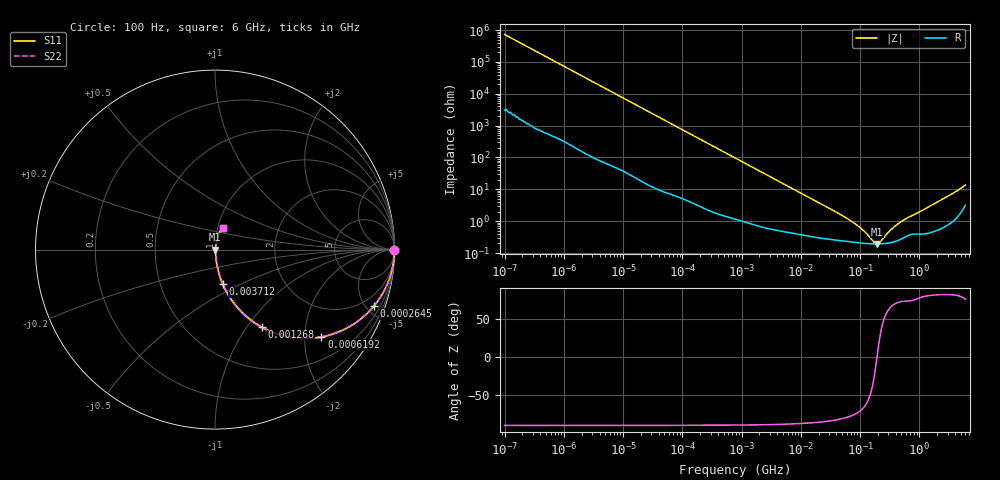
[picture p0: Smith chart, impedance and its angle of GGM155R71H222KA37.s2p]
!Murata Part Number: GGM155R71H222KA37
!These Parameters are Measured in Series Mode Connection
!Data Generated on Mar 13, 2026
!  o--ll--o
!Port1  Port2
!  o------o
!Operation Temp=25[degC], DC Bias Voltage=0[V]
!Freq. Start=100[Hz] Stop=6[GHz] 401[Steps]
# Hz S RI R 50
!Freq.(Hz) S11(Real) S11(Imag) S21(Real) S21(Imag) S12(Real) S12(Imag) S22(Real) S22(Imag)
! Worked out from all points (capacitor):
!   401 points, 100 Hz to 6 GHz, reference 50 ohm
!   read as one part in series: C = 2.18 nF near 109 Hz
!   lowest |Z| = 193 mohm at 190.9 MHz (marker M1)
!   series resonance near 192.9 MHz, so ESL is about 310 pH
!   S11 on the Smith chart (normalised r, x): 100 Hz: open; 264.5 kHz: 1.05, -5.64; 619.2 kHz: 1.03, -2.42; 1.268 MHz: 1.02, -1.19; 3.712 MHz: 1.01, -0.41; 6 GHz: 1.06, +0.27
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100  1 -0.000137  6e-07 0.000137  6e-07 0.000137  1 -0.000137
2008  1 -0.00274  1.9e-05 0.00274  1.9e-05 0.00274  1 -0.00274
40335  0.9968 -0.0543  0.00324 0.0543  0.00324 0.0543  0.9968 -0.0543
108014  0.9783 -0.1422  0.0217 0.1422  0.0217 0.1422  0.9783 -0.1422
264476  0.8863 -0.3135  0.1137 0.3135  0.1137 0.3135  0.8863 -0.3135
395726  0.7786 -0.4107  0.2214 0.4107  0.2214 0.4107  0.7786 -0.4107
619225  0.5924 -0.486  0.4076 0.486  0.4076 0.486  0.5924 -0.486
774597  0.4834 -0.4938  0.5166 0.4938  0.5166 0.4938  0.4834 -0.4938
1267578  0.2632 -0.433  0.7368 0.433  0.7368 0.433  0.2632 -0.433
2074311  0.1212 -0.3173  0.8788 0.3173  0.8788 0.3173  0.1212 -0.3173
3712478  0.0445 -0.1938  0.9555 0.1938  0.9555 0.1938  0.0445 -0.1938
1.555665e7  0.00561 -0.0489  0.9944 0.0489  0.9944 0.0489  0.00561 -0.0489
7.797396e7  0.00225 -0.00862  0.9977 0.00862  0.9977 0.00862  0.00225 -0.00862
1.166697e8  0.00203 -0.00443  0.998 0.00443  0.998 0.00443  0.00203 -0.00443
1.745687e8  0.00193 -0.000854  0.9981 0.000854  0.9981 0.000854  0.00193 -0.000854
1.909225e8  0.00192 -8.61e-05  0.9981 8.61e-05  0.9981 8.61e-05  0.00192 -8.61e-05
2.183701e8  0.00194 0.00107  0.9981 -0.00107  0.9981 -0.00107  0.00194 0.00107
3.124326e8  0.0021 0.00432  0.9979 -0.00432  0.9979 -0.00432  0.0021 0.00432
4.087225e8  0.00242 0.00707  0.9976 -0.00707  0.9976 -0.00707  0.00242 0.00707
5.59173e8  0.00318 0.0107  0.9968 -0.0107  0.9968 -0.0107  0.00318 0.0107
2.34314e9  0.00788 0.0452  0.9921 -0.0452  0.9921 -0.0452  0.00788 0.0452
6e9  0.0467 0.1228  0.9533 -0.1228  0.9533 -0.1228  0.0467 0.1228
